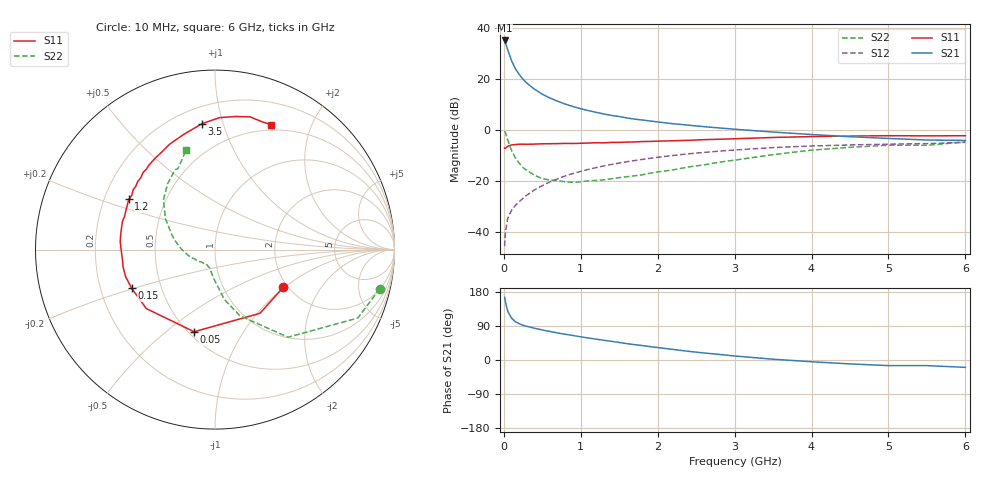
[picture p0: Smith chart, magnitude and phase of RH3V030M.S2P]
! SIEMENS Small Signal Semiconductors
! BFR106
! Si NPN RF Bipolar Junction Transistor in SOT23
! VCE = 3 V  IC = 30 mA
! Common Emitter S-Parameters:  August  1996
# GHz  S  MA  R  50
!  f  S11  S21  S12  S22
! GHz  MAG  ANG  MAG  ANG  MAG  ANG  MAG  ANG
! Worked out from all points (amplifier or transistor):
!   36 points, 10 MHz to 6 GHz, reference 50 ohm
!   highest |S21| = 35.0 dB at 10 MHz (marker M1)
!   |S21| within 3 dB of that: start of sweep to 43.41 MHz
!   unconditionally stable (mu >= 1): 293.2 MHz to 2.371 GHz; 5.36 GHz to 5.977 GHz
!   at 250 MHz: K = 0.96, MSG = 23.3 dB, |S12| = -26.9 dB
!   at 1.4 GHz: K = 1.06, MAG = 8.1 dB, |S12| = -13.6 dB
!   at 6 GHz: K = 1.00, MSG = 0.4 dB, |S12| = -5.0 dB
!   S11 on the Smith chart (normalised r, x): 10 MHz: 1.89, -0.98; 50 MHz: 0.53, -0.63; 150 MHz: 0.34, -0.20; 1.2 GHz: 0.30, +0.25; 3.5 GHz: 0.31, +0.85; 6 GHz: 0.44, +1.46
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0.01  0.4345 -29.0  56.45 165.6  0.0052 82.0  0.944 -13.3
0.02  0.4344 -54.8  52.02 153.8  0.0096 71.5  0.8823 -25.6
0.05  0.4722 -104.3  37.11 129.0  0.0183 59.3  0.6354 -50.2
0.1  0.5046 -139.4  22.69 110.4  0.0263 55.1  0.3927 -69.5
0.15  0.5118 -155.1  15.81 101.1  0.0327 58.1  0.2822 -79.4
0.2  0.5201 -163.0  12.15 95.7  0.0388 61.4  0.2206 -84.1
0.25  0.5213 -169.3  9.774 91.6  0.0454 63.3  0.1801 -89.3
0.3  0.5186 -173.1  8.185 88.8  0.0523 65.8  0.159 -93.0
0.4  0.523 -180.0  6.218 83.8  0.0662 67.4  0.1273 -99.4
0.5  0.5299 175.3  4.988 79.3  0.0802 68.4  0.1097 -104.3
0.6  0.5323 170.7  4.192 75.3  0.095 68.3  0.1031 -108.3
0.7  0.5349 166.6  3.62 71.3  0.1091 67.9  0.0997 -113.6
0.9  0.537 160.0  2.851 64.6  0.1387 66.3  0.0928 -122.3
1.1  0.5489 152.7  2.373 57.9  0.167 64.1  0.0994 -130.8
1.2  0.5562 149.7  2.196 55.0  0.181 63.0  0.1012 -135.1
1.6  0.5739 138.6  1.703 43.2  0.2358 57.4  0.1198 -150.9
2.2  0.6084 123.3  1.312 27.9  0.3132 48.5  0.1633 -172.9
2.8  0.6503 109.3  1.085 14.7  0.3804 39.0  0.2313 166.6
3.5  0.7051 95.9  0.901 2.1  0.4463 28.3  0.3247 148.2
4.5  0.7503 81.3  0.73 -10.3  0.5032 13.5  0.4522 125.7
5.5  0.7586 69.4  0.629 -14.8  0.5347 4.0  0.4959 114.6
6  0.7638 65.7  0.618 -19.4  0.5649 -3.1  0.578 106.1
